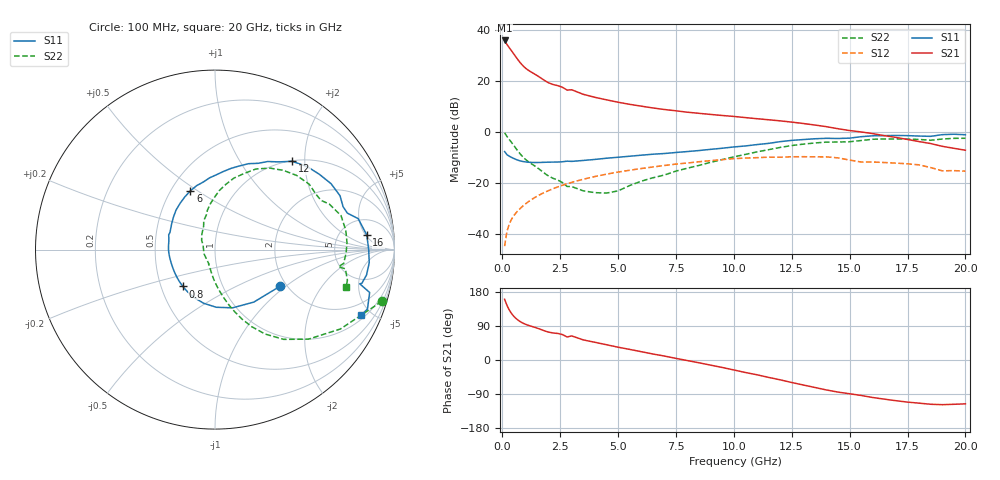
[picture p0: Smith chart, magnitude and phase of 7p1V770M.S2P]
! Infineon Technologies  Discrete & RF Semiconductors
! bfp620
! VCE =  1.7 V,  IC =  70 mA
! Common Emitter S-Parameters:  Sep 2002
# GHz  S  MA  R  50
!  f  S11  S21  S12  S22
! GHz  MAG  ANG  MAG  ANG  MAG  ANG  MAG  ANG
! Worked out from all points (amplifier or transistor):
!   59 points, 100 MHz to 20 GHz, reference 50 ohm
!   highest |S21| = 35.9 dB at 100 MHz (marker M1)
!   |S21| within 3 dB of that: start of sweep to 314.6 MHz
!   unconditionally stable (mu >= 1): 2.148 GHz to 2.229 GHz; 3.052 GHz to 9.888 GHz; 17.17 GHz to end of sweep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
!   at 1 GHz: K = 0.88, MSG = 26.6 dB, |S12| = -28.1 dB
!   at 5.5 GHz: K = 1.04, MAG = 11.7 dB, |S12| = -14.9 dB
!   at 20 GHz: K = 1.28, MAG = 0.9 dB, |S12| = -15.2 dB
!   S11 on the Smith chart (normalised r, x): 100 MHz: 1.86, -0.91; 800 MHz: 0.65, -0.29; 6 GHz: 0.62, +0.47; 12 GHz: 1.01, +1.73; 16 GHz: 9, +5; 20 GHz: 1.21, -4.32
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0.1  0.4173 -29.1  62.16 160.2  0.0059 78.4  0.9736 -17.2
0.2  0.3638 -53.5  52.06 144.4  0.0114 73.4  0.8274 -32.3
0.3  0.339 -73.1  44.92 132.0  0.0159 71.0  0.721 -43.8
0.4  0.3214 -88.7  38.96 122.5  0.0199 69.4  0.6295 -52.6
0.5  0.3057 -101.8  33.68 115.1  0.0234 68.2  0.5472 -59.3
0.6  0.2919 -113.1  29.07 109.2  0.0267 67.4  0.4747 -64.6
0.7  0.2808 -122.8  25.21 104.3  0.0299 66.8  0.4133 -68.9
0.8  0.2725 -131.1  22.12 100.3  0.0331 66.4  0.3634 -72.4
0.9  0.2665 -138.2  19.73 97.0  0.0363 66.0  0.3242 -75.4
1.1  0.2592 -149.0  16.54 92.0  0.0428 65.3  0.2702 -79.9
1.9  0.2584 -177.7  9.778 75.4  0.0689 60.4  0.1486 -95.2
2.8  0.2709 162.2  6.652 60.8  0.0982 53.0  0.0867 -114.7
3  0.2684 159.1  6.747 63.5  0.1044 51.1  0.0863 -113.4
3.5  0.2799 150.0  5.493 53.0  0.1204 46.4  0.0711 -131.2
6  0.3547 112.8  3.228 21.9  0.1945 21.9  0.1101 132.2
7  0.3824 99.7  2.777 10.4  0.223 12.1  0.1452 115.9
10.5  0.5377 63.4  1.927 -33.0  0.3116 -27.8  0.3675 80.7
12  0.6529 48.9  1.663 -52.3  0.3238 -45.5  0.5036 63.1
13.5  0.7436 29.6  1.38 -72.5  0.3295 -64.3  0.6151 42.1
16  0.8495 5.5  0.937 -99.0  0.2608 -88.2  0.7272 15.1
17  0.8625 -4.9  0.79 -107.4  0.2481 -96.1  0.7364 3.0
20  0.8915 -24.3  0.444 -115.7  0.1728 -105.9  0.76 -15.9
